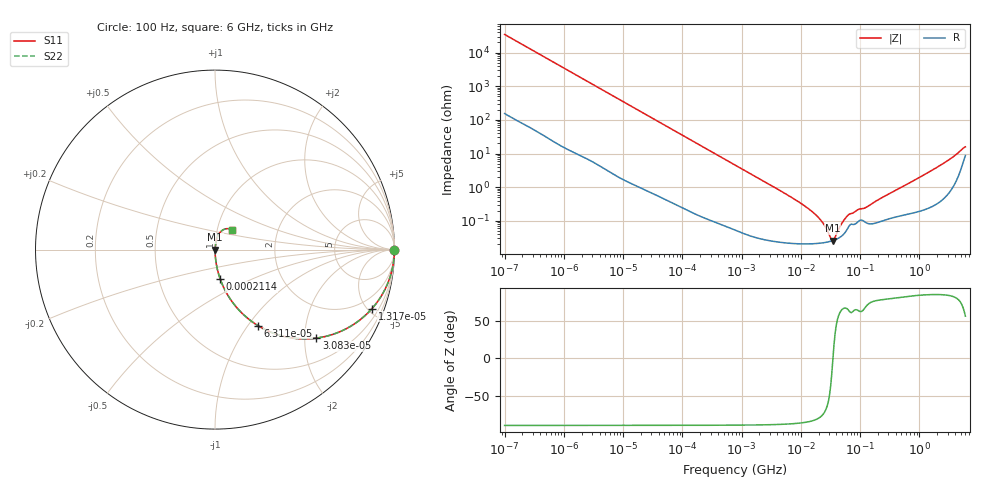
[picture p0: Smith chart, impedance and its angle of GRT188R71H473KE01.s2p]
!Murata Part Number: GRT188R71H473KE01
!These Parameters are Measured in Series Mode Connection
!Data Generated on Jun 19, 2026
!  o--ll--o
!Port1  Port2
!  o------o
!Operation Temp=25[degC], DC Bias Voltage=0[V]
!Freq. Start=100[Hz] Stop=6[GHz] 401[Steps]
# Hz S RI R 50
!Freq.(Hz) S11(Real) S11(Imag) S21(Real) S21(Imag) S12(Real) S12(Imag) S22(Real) S22(Imag)
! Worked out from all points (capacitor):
!   401 points, 100 Hz to 6 GHz, reference 50 ohm
!   read as one part in series: C = 46 nF near 109 Hz
!   lowest |Z| = 25.8 mohm at 34.83 MHz (marker M1)
!   series resonance near 34.85 MHz, so ESL is about 450 pH
!   S11 on the Smith chart (normalised r, x): 100 Hz: open; 13.17 kHz: 1.03, -5.32; 30.83 kHz: 1.01, -2.28; 63.12 kHz: 1.01, -1.12; 211.4 kHz: 1.00, -0.33; 6 GHz: 1.17, +0.26
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100  1 -0.00289  2.13e-05 0.00289  2.13e-05 0.00289  1 -0.00289
2008  0.9964 -0.0574  0.00359 0.0574  0.00359 0.0574  0.9964 -0.0574
5378  0.9762 -0.1501  0.0238 0.1501  0.0238 0.1501  0.9762 -0.1501
13169  0.875 -0.3283  0.125 0.3283  0.125 0.3283  0.875 -0.3283
30832  0.5645 -0.4929  0.4355 0.4929  0.4355 0.4929  0.5645 -0.4929
40335  0.4323 -0.4924  0.5677 0.4924  0.5677 0.4924  0.4323 -0.4924
63115  0.239 -0.4232  0.761 0.4232  0.761 0.4232  0.239 -0.4232
108014  0.0982 -0.2941  0.9018 0.2941  0.9018 0.2941  0.0982 -0.2941
211427  0.0285 -0.1624  0.9715 0.1624  0.9715 0.1624  0.0285 -0.1624
774597  0.00264 -0.0458  0.9974 0.0458  0.9974 0.0458  0.00264 -0.0458
6644369  0.000241 -0.00521  0.9998 0.00521  0.9998 0.00521  0.000241 -0.00521
1.555665e7  0.000211 -0.00186  0.9998 0.00186  0.9998 0.00186  0.000211 -0.00186
2.225763e7  0.000219 -0.000964  0.9998 0.000964  0.9998 0.000964  0.000219 -0.000964
3.184506e7  0.000246 -0.000189  0.9998 0.000189  0.9998 0.000189  0.000246 -0.000189
3.482834e7  0.000258 -1.5e-06  0.9997 1.5e-06  0.9997 1.5e-06  0.000258 -1.5e-06
3.80911e7  0.000273 0.000188  0.9997 -0.000188  0.9997 -0.000188  0.000273 0.000188
4.983056e7  0.000362 0.000789  0.9996 -0.000789  0.9996 -0.000789  0.000362 0.000789
6.233367e7  0.000609 0.00132  0.9994 -0.00132  0.9994 -0.00132  0.000609 0.00132
1.275994e8  0.000874 0.00237  0.9991 -0.00237  0.9991 -0.00237  0.000874 0.00237
3.124326e8  0.00119 0.00629  0.9988 -0.00629  0.9988 -0.00629  0.00119 0.00629
1.95892e9  0.00455 0.0378  0.9954 -0.0378  0.9954 -0.0378  0.00455 0.0378
6e9  0.0934 0.1096  0.9066 -0.1096  0.9066 -0.1096  0.0934 0.1096
